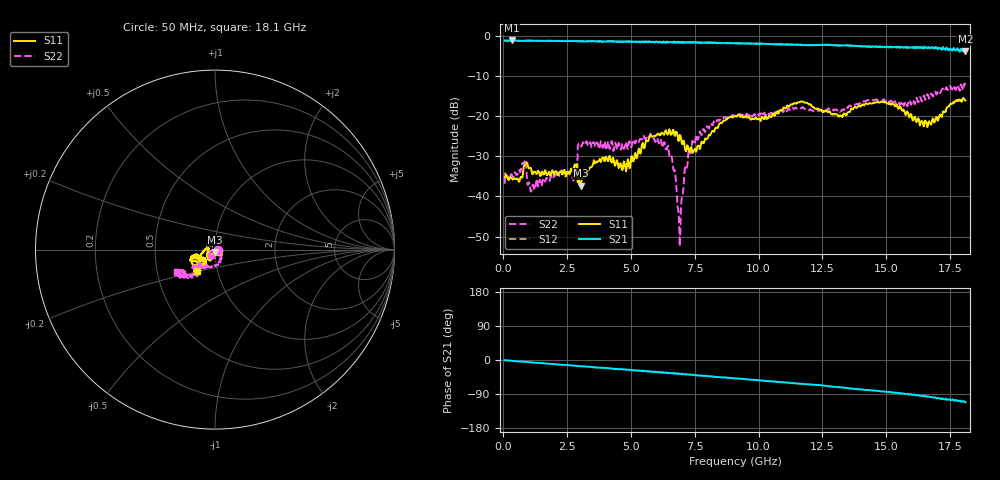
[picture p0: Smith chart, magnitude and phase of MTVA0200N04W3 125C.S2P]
! Network Analyzer HP8720D.06.14 Serial No. US36140669
! 17 Jan 2005  13:10:11
! Frequency  S11  S21  S12  S22
# HZ  S  DB R 50
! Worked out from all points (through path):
!   801 points, 50 MHz to 18.1 GHz, reference 50 ohm
!   highest |S21| = -1.21 dB at 320.8 MHz (marker M1); lowest = -3.9 dB at 18.1 GHz (marker M2)
!   group delay of S21, straight-line fit = 16.1 ps
!   lowest |S11| = -37.3 dB at 3.028 GHz (marker M3), VSWR 1.03, Z = 50.1 - j1.36 ohm
!   |S11| at or under -10 dB: start of sweep to end of sweep
!   |S22| runs from -52.4 to -11.9 dB; largest |S21 - S12| = 0.032
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5e7  -35.21 -18.3  -1.23 -0.6  -1.26 -1.0  -36.85 -4.8
3.2075e8  -35.36 -21.1  -1.21 -2.0  -1.21 -2.4  -34.44 -27.6
7.945625e8  -32.92 -9.5  -1.32 -4.5  -1.27 -4.9  -31.90 -57.9
1.155562e9  -34.48 -45.3  -1.28 -6.6  -1.28 -6.9  -37.11 -72.5
2.351375e9  -33.81 -60.5  -1.38 -12.8  -1.36 -13.1  -34.32 -101.9
2.734938e9  -33.83 -62.7  -1.36 -15.0  -1.38 -15.4  -36.08 -116.0
3.02825e9  -37.30 -85.4  -1.43 -16.5  -1.44 -17.0  -27.44 -98.7
3.073375e9  -35.64 -83.0  -1.41 -16.4  -1.38 -16.8  -27.30 -96.7
3.8405e9  -30.96 -76.8  -1.46 -20.6  -1.40 -20.9  -26.68 -118.2
4.878375e9  -30.75 -105.8  -1.57 -25.5  -1.52 -26.1  -28.25 -105.1
6.074188e9  -24.49 -123.1  -1.71 -32.6  -1.70 -32.9  -26.52 -130.9
6.63825e9  -23.46 -119.8  -1.70 -35.1  -1.68 -35.8  -32.12 -161.3
6.841312e9  -25.47 -136.1  -1.50 -36.4  -1.58 -36.4  -43.04 -165.2
6.909e9  -24.70 -135.1  -1.58 -36.3  -1.61 -37.4  -52.38 105.5
7.17975e9  -28.13 -155.2  -1.71 -37.4  -1.63 -38.1  -32.84 -25.6
7.473062e9  -28.45 174.8  -1.59 -39.4  -1.65 -40.2  -26.96 -45.2
9.075e9  -20.06 -146.9  -1.91 -48.6  -1.94 -49.0  -20.00 -109.8
1.209838e10  -17.59 -151.4  -2.32 -65.2  -2.34 -65.5  -18.61 -139.2
1.320394e10  -19.84 -150.1  -2.45 -72.1  -2.42 -72.5  -18.94 -134.1
1.509919e10  -16.91 -140.2  -2.93 -84.5  -2.88 -85.4  -16.40 -142.8
1.667856e10  -21.30 -142.1  -2.98 -97.1  -3.06 -98.7  -15.65 -127.8
1.81e10  -16.15 -130.3  -3.89 -111.4  -3.69 -112.9  -12.27 -149.5
